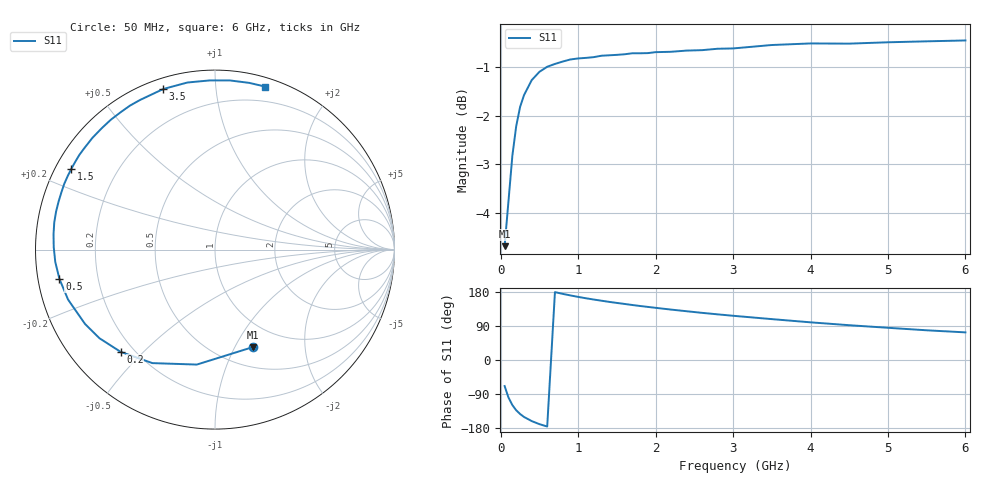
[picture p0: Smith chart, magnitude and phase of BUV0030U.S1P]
! Infineon Technologies  Discrete & RF Semiconductors
! BB 833
! Si Tuning Diode in SOD323
! VR =
! S-Parameters:  June  1999
# GHz  S  MA  R  50
!  f  S11
! GHz  MAG  ANG
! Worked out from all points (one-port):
!   34 points, 50 MHz to 6 GHz, reference 50 ohm
!   lowest |S11| = -4.7 dB at 50 MHz (marker M1), VSWR 3.79, Z = 36 - j59.2 ohm
!   |S11| at or under -10 dB: nowhere
!   S11 on the Smith chart (normalised r, x): 50 MHz: 0.72, -1.18; 200 MHz: 0.15, -0.43; 500 MHz: 0.06, -0.09; 1.5 GHz: 0.05, +0.26; 3.5 GHz: 0.05, +0.73; 6 GHz: 0.07, +1.35
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0.05  0.5827 -68.8
0.1  0.6486 -99.0
0.15  0.7224 -118.9
0.2  0.7752 -132.7
0.25  0.8113 -142.5
0.3  0.8343 -150.2
0.4  0.8647 -161.2
0.5  0.882 -169.3
0.6  0.8926 -175.6
0.7  0.8986 179.1
0.8  0.9038 174.5
0.9  0.9083 170.4
1.1  0.9117 162.9
1.3  0.9163 156.5
1.5  0.9182 150.6
1.6  0.9196 147.9
1.8  0.9217 142.5
2  0.9242 137.7
2.2  0.925 133.0
2.4  0.9276 128.7
2.8  0.9317 120.5
3  0.9324 116.7
3.5  0.94 107.9
4  0.9435 99.4
4.5  0.9431 91.8
5  0.9461 85.0
5.5  0.9483 78.4
6  0.9502 72.9
